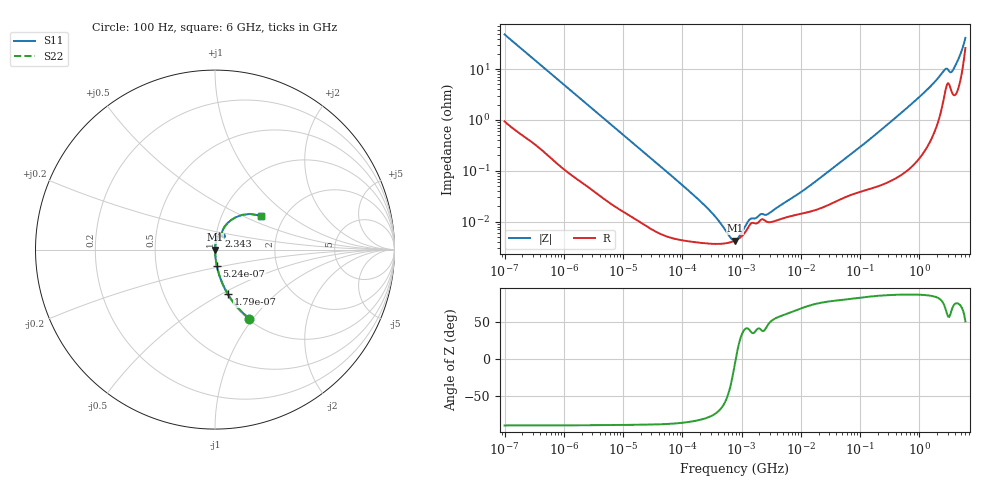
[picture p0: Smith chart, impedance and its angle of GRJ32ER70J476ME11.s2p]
!Murata Part Number: GRJ32ER70J476ME11
!These Parameters are Measured in Series Mode Connection
!Data Generated on Jun 19, 2026
!  o--ll--o
!Port1  Port2
!  o------o
!Operation Temp=25[degC], DC Bias Voltage=0[V]
!Freq. Start=100[Hz] Stop=6[GHz] 401[Steps]
# Hz S RI R 50
!Freq.(Hz) S11(Real) S11(Imag) S21(Real) S21(Imag) S12(Real) S12(Imag) S22(Real) S22(Imag)
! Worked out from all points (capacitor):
!   401 points, 100 Hz to 6 GHz, reference 50 ohm
!   read as one part in series: C = 33 uF near 109 Hz
!   lowest |Z| = 4.25 mohm at 774.6 kHz (marker M1)
!   series resonance near 796.9 kHz, so ESL is about 1.2 nH
!   S11 on the Smith chart (normalised r, x): 100 Hz: 1.02, -0.96; 179 Hz: 1.01, -0.54; 524 Hz: 1.00, -0.19; 2.343 GHz: 1.03, +0.16; 6 GHz: 1.52, +0.64
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100  0.192 -0.3842  0.808 0.3842  0.808 0.3842  0.192 -0.3842
179  0.0722 -0.2489  0.9278 0.2489  0.9278 0.2489  0.0722 -0.2489
524  0.0107 -0.0924  0.9893 0.0924  0.9893 0.0924  0.0107 -0.0924
2008  0.0012 -0.0248  0.9988 0.0248  0.9988 0.0248  0.0012 -0.0248
40335  6.07e-05 -0.00129  0.9999 0.00129  0.9999 0.00129  6.07e-05 -0.00129
184852  3.88e-05 -0.000273  1 0.000273  1 0.000273  3.88e-05 -0.000273
413847  3.64e-05 -9.6e-05  1 9.6e-05  1 9.6e-05  3.64e-05 -9.6e-05
473344  3.68e-05 -7.46e-05  1 7.46e-05  1 7.46e-05  3.68e-05 -7.46e-05
774597  4.23e-05 -3.9e-06  1 3.9e-06  1 3.9e-06  4.23e-05 -3.9e-06
1212075  6.76e-05 5.98e-05  0.9999 -5.98e-05  0.9999 -5.98e-05  6.76e-05 5.98e-05
2074311  0.000106 9e-05  0.9999 -9e-05  0.9999 -9e-05  0.000106 9e-05
2837864  9.74e-05 0.000104  0.9999 -0.000104  0.9999 -0.000104  9.74e-05 0.000104
1.555665e7  0.000162 0.000526  0.9998 -0.000526  0.9998 -0.000526  0.000162 0.000526
9.326766e7  0.000382 0.00271  0.9996 -0.00271  0.9996 -0.00271  0.000382 0.00271
3.124326e8  0.000686 0.00869  0.9993 -0.00869  0.9993 -0.00869  0.000686 0.00869
1.197065e9  0.00348 0.034  0.9965 -0.034  0.9965 -0.034  0.00348 0.034
2.34314e9  0.0208 0.0754  0.9792 -0.0754  0.9792 -0.0754  0.0208 0.0754
2.802721e9  0.0468 0.0852  0.9532 -0.0852  0.9532 -0.0852  0.0468 0.0852
3.352442e9  0.0458 0.0686  0.9542 -0.0686  0.9542 -0.0686  0.0458 0.0686
3.666503e9  0.0383 0.0819  0.9617 -0.0819  0.9617 -0.0819  0.0383 0.0819
4.796499e9  0.0742 0.1516  0.9258 -0.1516  0.9258 -0.1516  0.0742 0.1516
6e9  0.2544 0.1889  0.7456 -0.1889  0.7456 -0.1889  0.2544 0.1889
